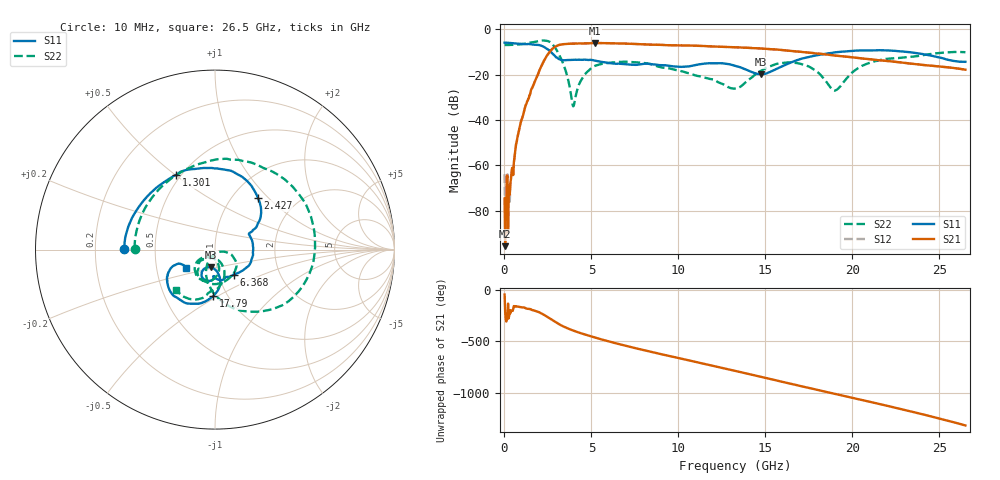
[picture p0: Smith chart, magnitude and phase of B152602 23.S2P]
!  2-Port S-parameters saved by WinCal
! VAR MeasName=S-Parameters (CALIBRATED_DATA) read from VNA (N5242A)
! VAR MeasDate=2016-1-5 16:28:35
! VAR NAME=B152602 23
! VAR FILENAME=B152602 23.S2P
! VAR DATE=2016-1-5 16:28:35
! VAR PHYS_PORTS=1,2
# Hz S DB R 50
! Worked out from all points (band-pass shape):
!   801 points, 10 MHz to 26.5 GHz, reference 50 ohm
!   highest |S21| = -6.08 dB at 5.209 GHz (marker M1); lowest = -95.6 dB at 43.11 MHz (marker M2)
!   |S21| within 3 dB of the highest: 2.701 GHz to 15.85 GHz (13.15 GHz wide, 142 % of centre)
!   lowest |S11| = -19.9 dB at 14.75 GHz (marker M3), VSWR 1.23, Z = 46.9 - j9.39 ohm
!   |S11| at or under -10 dB: 2.672 GHz to 19.25 GHz (16.57 GHz wide, 151 % of centre); 23.14 GHz to end of sweep
!   |S22| runs from -34.0 to -4.9 dB; largest |S21 - S12| = 0.0031
!   S11 on the Smith chart (normalised r, x): 10 MHz: 0.33, +0.00; 1.301 GHz: 0.47, +0.50; 2.427 GHz: 1.30, +0.87; 6.368 GHz: 1.18, -0.34; 17.79 GHz: 0.86, -0.48; 26.5 GHz: 0.71, -0.15
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1e7  -5.93 179.4  -74.58 -43.9  -63.94 119.3  -6.97 179.4
4.31125e7  -5.92 177.8  -95.62 144.8  -83.48 156.4  -6.97 177.4
1.755625e8  -5.96 170.9  -64.70 80.3  -63.97 83.4  -6.95 169.2
3.41125e8  -6.07 162.6  -67.89 133.4  -67.26 139.3  -6.92 159.0
8.047e8  -6.39 140.7  -45.64 -162.3  -45.62 -162.5  -6.75 130.2
1.301388e9  -6.58 117.5  -31.78 178.1  -31.78 178.0  -6.23 97.5
2.427212e9  -8.54 50.4  -11.83 102.8  -11.82 102.8  -5.11 -2.4
2.824562e9  -11.18 30.7  -8.18 59.9  -8.17 59.9  -7.20 -51.6
3.288138e9  -13.57 25.4  -6.70 14.1  -6.70 14.2  -13.56 -97.7
3.950388e9  -13.43 12.0  -6.33 -34.1  -6.33 -34.1  -33.97 -68.4
4.447075e9  -13.49 -3.5  -6.28 -63.4  -6.28 -63.3  -22.01 -14.8
5.208662e9  -13.86 -29.1  -6.08 -102.5  -6.07 -102.4  -16.13 -41.3
6.3676e9  -15.18 -53.4  -6.23 -156.6  -6.22 -156.6  -14.59 -77.9
8.851038e9  -15.76 -86.9  -6.84 102.0  -6.81 101.9  -16.48 -130.0
1.116891e10  -15.51 -94.0  -7.32 13.1  -7.28 13.2  -20.67 -141.3
1.3255e10  -16.10 -118.5  -7.94 -66.4  -7.92 -66.6  -26.18 -107.7
1.474506e10  -19.87 -102.7  -8.52 -124.9  -8.48 -124.9  -18.30 -79.7
1.769208e10  -11.86 -91.4  -10.47 119.5  -10.42 119.7  -17.26 -142.3
1.779141e10  -11.71 -92.4  -10.57 115.7  -10.49 115.7  -17.76 -144.3
1.901658e10  -10.21 -104.8  -11.62 68.6  -11.55 68.4  -27.01 -104.9
2.209604e10  -9.36 -137.6  -14.08 -50.6  -14.02 -51.0  -12.98 -90.4
2.65e10  -14.37 -148.1  -17.83 121.8  -17.81 121.7  -10.13 -133.7
